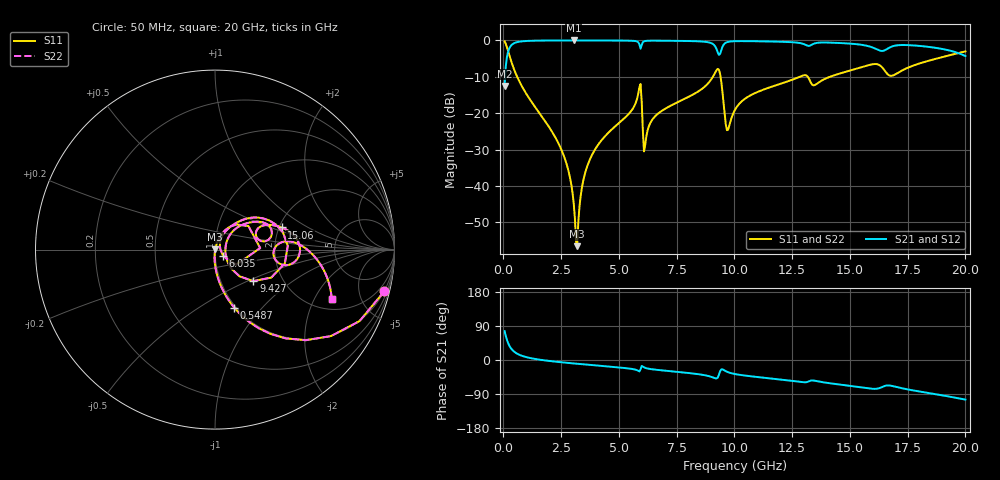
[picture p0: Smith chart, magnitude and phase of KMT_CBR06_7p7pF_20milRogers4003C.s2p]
! Data measured by Modelithics Inc. support@modelithics.com 813-866-6335
! KEMET CBR0603 7.7pF, Pad Width= 0.851mm, Pad Length= 0.64mm, Pad Gap= 0.62mm, 20mil Rogers 4003C substrate Data, January 2022
# hz S ma R 50
! 2 Port Network Data from SP1.SP block
! freq  magS11  angS11  magS21  angS21  magS12  angS12  magS22  angS22
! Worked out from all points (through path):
!   401 points, 50 MHz to 20 GHz, reference 50 ohm
!   highest |S21| = -0.01 dB at 3.042 GHz (marker M1); lowest = -12.5 dB at 50 MHz (marker M2)
!   group delay of S21, straight-line fit = 14.9 ps
!   lowest |S11| = -56.5 dB at 3.192 GHz (marker M3), VSWR 1.00, Z = 50.1 + j0.0649 ohm
!   |S11| at or under -10 dB: 594 MHz to 9.066 GHz (8.472 GHz wide, 175 % of centre); 9.398 GHz to 12.83 GHz (3.428 GHz wide, 30.8 % of centre); 13.18 GHz to 14.14 GHz (957.9 MHz wide, 7.01 % of centre)
!   |S22| runs from -56.5 to -0.3 dB; largest |S21 - S12| = 0
!   S11 on the Smith chart (normalised r, x): 50 MHz: 0.98, -8.11; 548.8 MHz: 0.98, -0.72; 6.035 GHz: 1.09, -0.08; 9.427 GHz: 1.42, -0.54; 15.06 GHz: 2.06, +0.60; 20 GHz: 2.52, -2.78
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5e7  0.9714 -13.9  0.237 76.1  0.237 76.1  0.9714 -13.9
2.495e8  0.6322 -51.5  0.774 38.4  0.774 38.4  0.6322 -51.5
5.4875e8  0.3409 -71.6  0.9393 18.2  0.9393 18.2  0.3409 -71.6
2.493875e9  0.0323 -94.0  0.9983 -5.9  0.9983 -5.9  0.0323 -94.0
2.843e9  0.01477 -93.5  0.9986 -8.0  0.9986 -8.0  0.01477 -93.5
3.0425e9  0.00575 -87.3  0.9987 -9.1  0.9987 -9.1  0.00575 -87.3
3.192125e9  0.001488 25.8  0.9987 -9.9  0.9987 -9.9  0.001488 25.8
3.391625e9  0.00927 71.2  0.9986 -11.0  0.9986 -11.0  0.00927 71.2
3.94025e9  0.03078 73.5  0.998 -14.0  0.998 -14.0  0.03078 73.5
5.8355e9  0.185 49.2  0.9436 -28.4  0.9436 -28.4  0.185 49.2
6.035e9  0.05829 -38.1  0.945 -17.5  0.945 -17.5  0.05829 -38.1
6.184625e9  0.0475 54.1  0.9871 -21.7  0.9871 -21.7  0.0475 54.1
6.73325e9  0.101 61.6  0.9915 -26.6  0.9915 -26.6  0.101 61.6
9.0275e9  0.3019 36.1  0.9079 -45.1  0.9079 -45.1  0.3019 36.1
9.4265e9  0.2769 -39.4  0.7291 -25.0  0.7291 -25.0  0.2769 -39.4
9.675875e9  0.05837 -9.3  0.9452 -30.9  0.9452 -30.9  0.05837 -9.3
1.0025e10  0.1113 43.9  0.9762 -37.1  0.9762 -37.1  0.1113 43.9
1.291775e10  0.325 25.2  0.9086 -58.2  0.9086 -58.2  0.325 25.2
1.336662e10  0.2465 13.5  0.8786 -53.9  0.8786 -53.9  0.2465 13.5
1.506238e10  0.3906 18.5  0.9008 -68.7  0.9008 -68.7  0.3906 18.5
1.670825e10  0.3301 -6.7  0.7951 -67.3  0.7951 -67.3  0.3301 -6.7
2e10  0.7067 -23.0  0.6092 -104.5  0.6092 -104.5  0.7067 -23.0
